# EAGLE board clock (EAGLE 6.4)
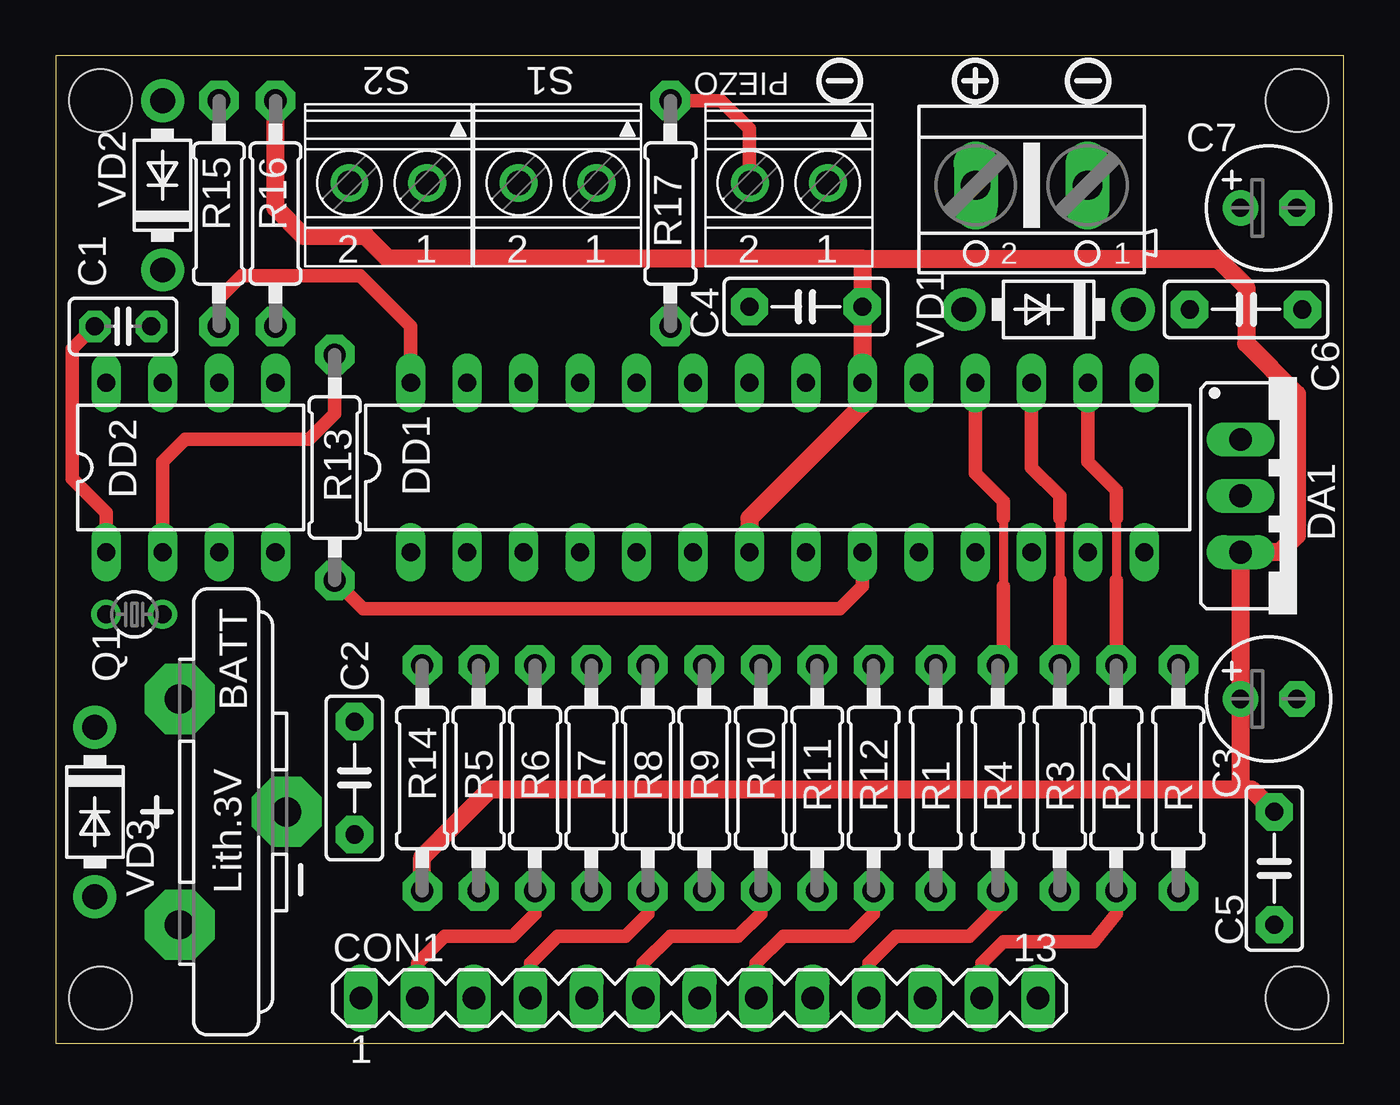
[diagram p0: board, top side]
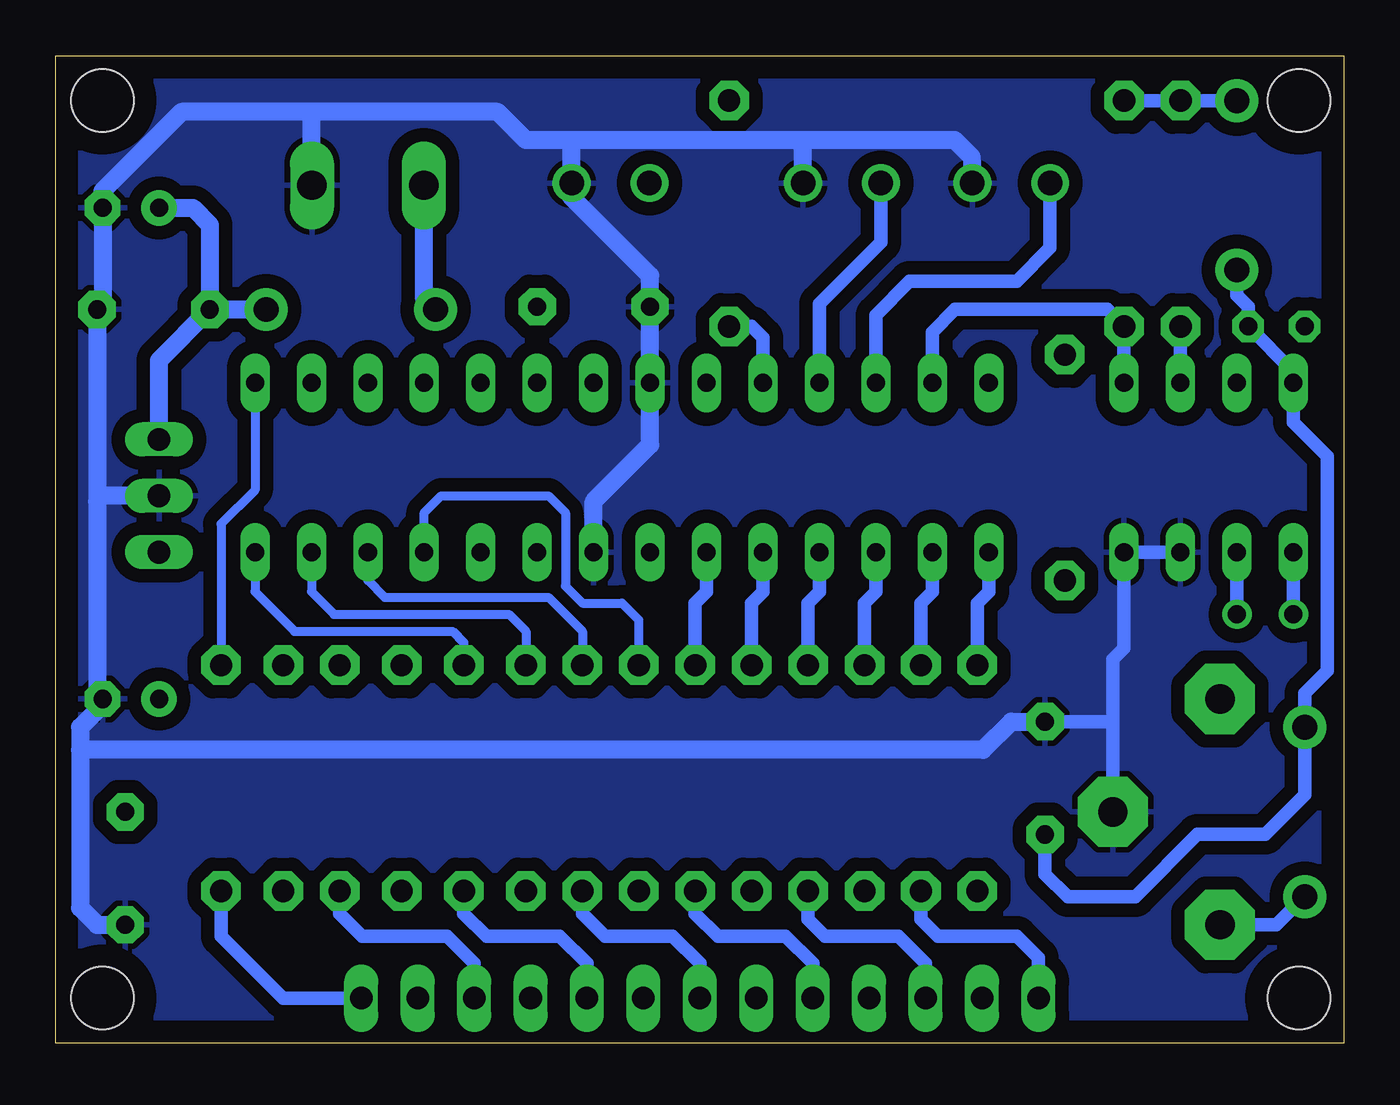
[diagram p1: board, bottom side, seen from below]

Size 57.99 x 44.44 mm. Coordinates in mm from the lower left corner, seen from the top.
Outline: 57.99,0 57.99,44.44 0,44.44 0,0 57.99,0
Copper layers (1*16): Top 0.035mm / dielectric 1.5mm / Bottom 0.035mm
Design rules "default": minimum track width 10mil, minimum drill 24mil, track to track 8mil, track to pad 8mil, pad to pad 8mil, via to via 8mil, smd to smd 8mil, copper to edge 40mil, drill to drill 8mil, minimum pad ring 10mil, minimum via ring 8mil, stop-mask expansion 4mil, vias tented up to drill 0mil, thermal gap 10mil
Holes 2.8 mm at 2.02,2.03 55.87,2.03 2.02,42.42 55.87,42.42

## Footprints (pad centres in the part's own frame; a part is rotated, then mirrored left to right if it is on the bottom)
AK500/2 = drill 1.321 long: 1 -2.515,0; 2 2.515,0
CR2032V = drill 1.321 pad 3.15 octagon: + -2.54,-5.08; +@1 -2.54,5.08; - 2.286,0
C025-025X050 = drill 0.813 pad 1.422 octagon: 1 -1.27,0; 2 1.27,0
C050-025X075 = drill 0.813 pad 1.676 octagon: 1 -2.54,0; 2 2.54,0
E2,5-6 = drill 0.813 pad 1.6: + -1.27,0 | drill 0.813 pad 1.6 octagon: - 1.27,0
MA13-1 = drill 1.016 long: 1 -15.24,0; 2 -12.7,0; 3 -10.16,0; 4 -7.62,0; 5 -5.08,0; 6 -2.54,0; 7 0,0; 8 2.54,0; 9 5.08,0; 10 7.62,0; 11 10.16,0; 12 12.7,0; 13 15.24,0
78XXS = drill 1.016 long: GND 0,-2.54; IN -2.54,-2.54; OUT 2.54,-2.54
DIL28-3 = drill 0.813 long: 1 -16.51,-3.81; 2 -13.97,-3.81; 3 -11.43,-3.81; 4 -8.89,-3.81; 5 -6.35,-3.81; 6 -3.81,-3.81; 7 -1.27,-3.81; 8 1.27,-3.81; 9 3.81,-3.81; 10 6.35,-3.81; 11 8.89,-3.81; 12 11.43,-3.81; 13 13.97,-3.81; 14 16.51,-3.81; 15 16.51,3.81; 16 13.97,3.81; 17 11.43,3.81; 18 8.89,3.81; 19 6.35,3.81; 20 3.81,3.81; 21 1.27,3.81; 22 -1.27,3.81; 23 -3.81,3.81; 24 -6.35,3.81; 25 -8.89,3.81; 26 -11.43,3.81; 27 -13.97,3.81; 28 -16.51,3.81
DIL08 = drill 0.813 long: 1 -3.81,-3.81; 2 -1.27,-3.81; 3 1.27,-3.81; 4 3.81,-3.81; 5 3.81,3.81; 6 1.27,3.81; 7 -1.27,3.81; 8 -3.81,3.81
TC26V = drill 0.813: 1 -1.27,0; 2 1.27,0
0207/10 = drill 1 pad 1.778 octagon: 1 -5.08,0; 2 5.08,0
DO41-10 = drill 1.118 pad 1.93: A 3.81,0; C -3.81,0
1751248 = drill 1.1 pad 1.7: 1 -1.75,-0.1; 2 1.75,-0.1

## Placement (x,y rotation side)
+12V  [AK500/2]  43.93,38.61 180 top
BATT  CR2032V  [CR2032V]  8.12,10.41 0 top
C1  [C025-025X050]  3.04,32.26 0 top
C2  100nF  [C050-025X075]  13.45,11.94 90 top
C3  220uF  [E2,5-6]  54.6,15.49 0 top
C4  100nF  [C050-025X075]  33.77,33.15 180 top
C5  100nF  [C050-025X075]  54.85,7.87 270 top
C6  100nF  [C050-025X075]  53.58,33.02 0 top
C7  220uF  [E2,5-6]  54.6,37.59 0 top
CON1  [MA13-1]  28.99,2.03 0 top
DA1  7805  [78XXS]  55.87,24.64 270 top
DD1  ATMEGA8  [DIL28-3]  32.5,25.91 0 top
DD2  PFC8583P  [DIL08]  6.09,25.91 0 top
Q1  [TC26V]  3.55,19.3 180 top
R  [0207/10]  50.54,11.94 90 top
R1  [0207/10]  39.61,11.94 90 top
R2  [0207/10]  47.74,11.94 90 top
R3  [0207/10]  45.2,11.94 90 top
R4  47  [0207/10]  42.41,11.94 90 top
R5  [0207/10]  19.04,11.94 90 top
R6  [0207/10]  21.58,11.94 90 top
R7  [0207/10]  24.12,11.94 90 top
R8  [0207/10]  26.66,11.94 90 top
R9  [0207/10]  29.2,11.94 90 top
R10  [0207/10]  31.74,11.94 90 top
R11  [0207/10]  34.28,11.94 90 top
R12  [0207/10]  36.82,11.94 90 top
R13  [0207/10]  12.56,25.91 270 top
R14  3,3k  [0207/10]  16.5,11.94 90 top
R15  [0207/10]  7.36,37.34 90 top
R16  [0207/10]  9.9,37.34 90 top
R17  [0207/10]  27.68,37.34 90 top
VD1  1N4007  [DO41-10]  44.69,33.02 180 top
VD2  1N4007  [DO41-10]  4.82,38.61 90 top
VD3  1N4007  [DO41-10]  1.77,10.41 270 top
X1  1751248  [1751248]  22.6,38.61 180 top
X2  1751248  [1751248]  14.98,38.61 180 top
X3  1751248  [1751248]  33.01,38.61 180 top

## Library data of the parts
+12V = con-ptr500; OC_FARNELL: unknown; OC_NEWARK: unknown
BATT = battery
C1-C7 R R1-R17 = rcl
CON1 = con-lstb; OC_FARNELL: unknown; OC_NEWARK: unknown
DA1 = v-reg
DD1 = avr-4
DD2 = micro-philips; OC_FARNELL: unknown; OC_NEWARK: unknown
Q1 = crystal; OC_FARNELL: unknown; OC_NEWARK: unknown
VD1-VD3 = diode
X1-X3 = con-phoenix-350; OC_FARNELL: unknown; OC_NEWARK: unknown

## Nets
32K: DD1.9 R13.2
+5V: C3.+ C4.1 C5.1 DA1.OUT DD1.7 DD1.20 R14.1 R15.2 R16.2 VD2.A
+12V: C6.1 C7.+ DA1.IN VD1.C
A: DD1.2 R5.2
A1: DD1.14 R1.2
A2: DD1.18 R4.2
A3: DD1.17 R3.2
A4: DD1.16 R2.2
A5: DD1.15 R.2
B: DD1.3 R6.2
C: DD1.4 R7.2
D: DD1.5 R8.2
DP: DD1.13 R12.2
E: DD1.6 R9.2
F: DD1.11 R10.2
G: DD1.12 R11.2
GND: +12V.1 BATT.- C2.2 C3.- C4.2 C5.2 C6.2 C7.- DA1.GND DD1.8 DD1.22 DD2.3 DD2.4 X1.1 X2.1 X3.1
N$1: CON1.1 R5.1
N$2: CON1.2 R6.1
N$3: CON1.3 R7.1
N$4: CON1.4 R8.1
N$5: CON1.5 R9.1
N$6: CON1.6 R10.1
N$7: CON1.7 R11.1
N$8: CON1.8 R12.1
N$9: CON1.9 R1.1
N$10: CON1.10 R4.1
N$11: CON1.11 R3.1
N$12: CON1.12 R2.1
N$13: CON1.13 R.1
N$14: R17.2 X3.2
N$22: BATT.+ VD3.A
N$23: DD1.1 R14.2
N$24: +12V.2 VD1.A
N$25: C1.1 DD2.1 Q1.2
N$26: DD2.2 Q1.1 R13.1
N$40: C1.2 C2.1 DD2.8 VD2.C VD3.C
PIEZO: DD1.24 R17.1
S1: DD1.25 X1.2
S2: DD1.26 X2.2
SCL: DD1.28 DD2.6 R15.1
SDA: DD1.27 DD2.5 R16.1

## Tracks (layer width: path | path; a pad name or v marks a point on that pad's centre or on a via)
32K
  Top 0.61: DD1.9 36.31,20.57 35.3,19.56 13.83,19.56 R13.2
+5V
  Top 0.813: DD1.7 31.23,23.62 36.31,28.7 DD1.20 C4.1 36.31,35.31 | R14.1 16.5,8.38 19.55,11.43 53.58,11.43 | 53.58,11.43 53.84,11.43 C5.1 | 36.31,35.31 52.31,35.31 53.58,34.04 53.58,31.5 55.87,29.21 55.87,22.86 55.11,22.1 DA1.OUT C3.+ 53.33,11.68 53.58,11.43 | 36.31,35.31 14.98,35.31 13.96,36.32 11.17,36.32 9.9,37.59 R16.2
  Bottom 0.61: VD2.A R15.2 R16.2
+12V
  Bottom 0.813: DA1.IN 53.33,30.73 C6.1 | C6.1 VD1.C | C7.+ 51.81,37.59 51.04,36.83 C6.1
A
  Bottom 0.61: R5.2 19.04,19.81 18.53,20.32 DD1.2
A1
  Bottom 0.406: DD1.14 49.01,20.32 47.23,18.54 40.12,18.54 39.61,18.03 R1.2
A2
  Top 0.406: 42.66,23.62 42.66,20.57
  Top 0.61: DD1.18 41.39,25.65 42.66,24.38 42.66,23.62 | 42.66,20.57 42.66,17.27 R4.2
A3
  Top 0.406: 45.2,23.62 45.2,20.83
  Top 0.61: DD1.17 43.93,25.91 45.2,24.64 45.2,23.62 | 45.2,20.83 R3.2
A4
  Top 0.406: 47.74,23.62 47.74,20.83
  Top 0.61: DD1.16 46.47,26.16 47.74,24.89 47.74,23.62 | 47.74,20.83 R2.2
A5
  Bottom 0.406: DD1.15 49.01,24.89 50.54,23.37 R.2
B
  Bottom 0.61: R6.2 21.58,19.81 21.07,20.32 DD1.3
C
  Bottom 0.61: R7.2 24.12,19.81 23.61,20.32 DD1.4
D
  Bottom 0.61: R8.2 26.66,19.81 26.15,20.32 DD1.5
DP
  Bottom 0.406: DD1.13 46.47,20.32 45.46,19.3 37.58,19.3 36.82,18.54 R12.2
E
  Bottom 0.61: R9.2 29.2,19.81 28.69,20.32 DD1.6
F
  Bottom 0.406: DD1.11 41.39,23.88 40.63,24.64 35.8,24.64 35.04,23.88 35.04,20.57 34.28,19.81 32.5,19.81 31.74,19.05 R10.2
G
  Bottom 0.406: DD1.12 43.93,20.83 43.17,20.07 35.8,20.07 34.28,18.54 R11.2
GND
  Bottom 0.61: DD2.3 DD2.4 9.9,17.78 10.4,17.27 10.4,14.48 | BATT.- 10.4,14.48 | C2.2 10.4,14.48
  Bottom 0.813: +12V.1 46.45,38.58 46.47,41.91 | 46.47,41.91 52.31,41.91 55.87,38.35 C7.- 55.87,33.53 C6.2 56.12,24.38 | 56.12,24.38 56.12,15.75 C3.- 55.87,15.24 56.89,14.22 56.89,13.21 | 56.89,13.21 56.89,6.1 56.12,5.33 C5.2 | DA1.GND 55.87,24.64 56.12,24.38 | DD1.8 33.77,24.38 31.23,26.92 DD1.22 C4.2 31.23,34.54 34.79,38.1 34.79,38.68 X3.1 34.76,40.61 34.79,40.64 | X2.1 16.73,39.6 16.75,39.88 17.52,40.64 24.63,40.64 | 24.63,40.64 34.79,40.64 | 34.79,40.64 36.82,40.64 38.09,41.91 46.47,41.91 | X1.1 24.35,40.36 24.63,40.64 | 56.89,13.21 16.25,13.21 14.98,14.48 C2.2
  pour Bottom (isolate 0.61): -0.77,45.21 59.17,45.21 59.43,-1.02 -0.77,-1.02
N$1
  Bottom 0.61: CON1.1 13.75,3.85 14.72,4.83 18.28,4.83 19.04,5.59 R5.1
N$2
  Top 0.61: CON1.2 16.29,3.6 17.52,4.83 20.56,4.83 21.58,5.84 R6.1
N$3
  Bottom 0.61: CON1.3 18.83,3.6 20.06,4.83 23.36,4.83 24.12,5.59 R7.1
N$4
  Top 0.61: CON1.4 21.37,3.6 22.6,4.83 25.64,4.83 26.66,5.84 R8.1
N$5
  Bottom 0.61: CON1.5 23.91,3.6 25.14,4.83 28.18,4.83 29.2,5.84 R9.1
N$6
  Top 0.61: CON1.6 26.45,3.6 27.68,4.83 30.72,4.83 31.74,5.84 R10.1
N$7
  Bottom 0.61: CON1.7 28.99,3.6 30.22,4.83 33.26,4.83 34.28,5.84 R11.1
N$8
  Top 0.61: R12.1 36.82,5.84 35.8,4.83 32.76,4.83 31.53,3.6 CON1.8
N$9
  Bottom 0.61: CON1.9 34.07,3.6 35.3,4.83 38.6,4.83 39.61,5.84 R1.1
N$10
  Top 0.61: CON1.10 36.61,3.6 37.84,4.83 41.14,4.83 42.41,6.1 R4.1
N$11
  Bottom 0.61: CON1.11 39.15,3.6 40.38,4.83 44.19,4.83 45.2,5.84 R3.1
N$12
  Top 0.61: CON1.12 41.69,3.6 42.66,4.57 46.73,4.57 47.74,5.84 R2.1
N$13
  Bottom 0.61: CON1.13 47.74,2.03 50.54,4.83 R.1
N$14
  Top 0.61: R17.2 29.96,42.42 31.23,41.15 31.23,38.74 X3.2
N$22
  Bottom 0.61: VD3.A 3.04,5.33 BATT.+
N$23
  Bottom 0.61: R14.2 16.5,19.81 15.99,20.32 DD1.1
N$24
  Bottom 0.813: +12V.2 41.42,33.55 VD1.A
N$25
  Top 0.61: C1.1 0.75,31.24 0.75,25.4 2.28,23.88 DD2.1
  Bottom 0.61: DD2.1 Q1.2
N$26
  Top 0.61: R13.1 12.56,28.32 11.42,27.18 5.83,27.18 4.82,26.16 DD2.2
  Bottom 0.61: DD2.2 Q1.1
N$40
  Bottom 0.61: VD2.C 4.82,33.66 4.31,33.15 C1.2 2.28,30.23 DD2.8 2.28,27.94 0.75,26.42 0.75,16.76 1.77,15.75 VD3.C 1.77,11.18 3.55,9.4 6.59,9.4 9.39,6.6 12.44,6.6 13.45,7.62 C2.1
PIEZO
  Bottom 0.61: R17.1 26.66,32.26 26.15,31.75 DD1.24
S1
  Bottom 0.61: X1.2 20.85,36.04 23.61,33.27 DD1.25
S2
  Bottom 0.61: X2.2 13.23,35.79 14.72,34.29 19.55,34.29 21.07,32.77 DD1.26
SCL
  Top 0.61: DD1.28 15.99,32.26 13.71,34.54 8.37,34.54 7.36,33.53 R15.1
  Bottom 0.61: DD2.6 R15.1
SDA
  Bottom 0.61: DD2.5 R16.1 10.66,33.02 17.52,33.02 18.53,32 DD1.27

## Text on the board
tNames: S2 | S1 | PIEZO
